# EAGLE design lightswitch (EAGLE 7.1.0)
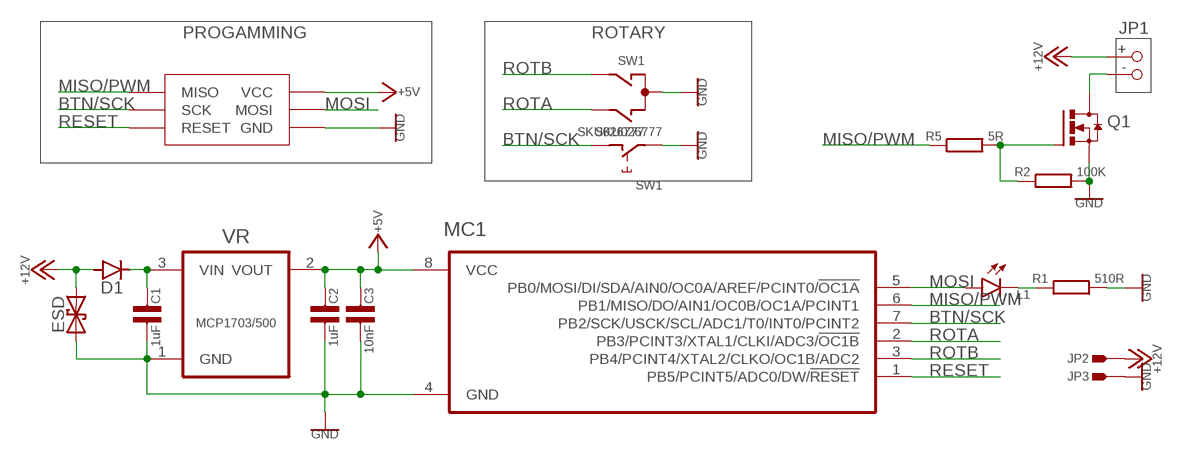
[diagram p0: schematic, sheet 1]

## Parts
C1  1uF  C-EU0603  [0603]
C2  1uF  C-EU0603  [0603]
C3  10nF  C-EU0603  [0603]
D1  DIODE0603  [0603-DIODE]
ESD  ESDSUPPRESSOR0603  [0603]
JP1  PINHD-1X2LED-STRIP  [CON-LEDSTRIP]
JP2  PINHD-1X11.5MM2  [1X01-HUGE]
JP3  PINHD-1X11.5MM2  [1X01-HUGE]
L1  LED0603  [0603-DIODE]
MC1  ATTINY85SOIC  [SOIC8-WIDE]
Q1  MOSFET-NCHSOT-23  [SOT23]
R1  510R  R-EU0603  [0603]
R2  100K  R-EU0603  [0603]
R5  5R  R-EU0603  [0603]
SW1  SKU026777  [SKU026777]
U$1  AVRISPTAG-CONNECT  [TAG-CONNECT-2030NL]
VR  MCP1703/500  MCP1703SOT23  [SOT23]

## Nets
+12V: D1.2(A) ESD.2 JP1.+ JP2.P$1
BTN/SCK: MC1.7(PB2/SCK/USCK/SCL/ADC1/T0/INT0/PCINT2) SW1.D U$1.3(SCK)
GND: C1.1 C2.1 C3.1 ESD.1 JP3.P$1 MC1.4(GND) Q1.2(S) R1.2 R2.2 SW1.C SW1.E U$1.6(GND) VR.1(GND)
MISO/PWM: MC1.6(PB1/MISO/DO/AIN1/OC0B/OC1A/PCINT1) R5.1 U$1.1(MISO)
MOSI: L1.2(A) MC1.5(PB0/MOSI/DI/SDA/AIN0/OC0A/AREF/PCINT0/!OC1A) U$1.4(MOSI)
N$1: C1.2 D1.1(K) VR.3(VIN)
N$2: L1.1(C) R1.1
OUT1: JP1.- Q1.3(D)
OWM: Q1.1(G) R2.1 R5.2
RESET: MC1.1(PB5/PCINT5/ADC0/DW/!RESET) U$1.5(RESET)
ROTA: MC1.2(PB3/PCINT3/XTAL1/CLKI/ADC3/!OC1B) SW1.B
ROTB: MC1.3(PB4/PCINT4/XTAL2/CLKO/OC1B/ADC2) SW1.A
VCC: C2.2 C3.2 MC1.8(VCC) U$1.2(VCC) VR.2(VOUT) ; supply symbol labelled +5V
Unconnected: SW1.GND1(G) SW1.GND2(G)

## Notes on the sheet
- PROGAMMING | ROTARY

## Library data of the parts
C1-C3 = MikesParts:C-EU
D1 = MikesParts:DIODE
ESD = MikesParts:ESDSUPPRESSOR: ESD Suppressor
JP1 = MikesParts:PINHD-1X2: PIN HEADER
JP2 JP3 = MikesParts:PINHD-1X1: PIN HEADER
L1 = MikesParts:LED: LED
MC1 = MikesParts:ATTINY85: 8-bit Microcontroller with In-System Programmable Flash; MPN: ATTINY85-20SU; OC_FARNELL: 1455164; OC_NEWARK: 58M3797; PACKAGE: SOIC-8; SUPPLIER: Atmel
Q1 = MikesParts:MOSFET-NCH: MOSFET N-Channel, eg BSS138, BUK7Y13, FDN335N
R1 R2 R5 = MikesParts:R-EU: resistor
SW1 = MikesParts:SKU026777: ALPS rotary Encoder EC12E series with switch; MPN: EC12E2424407; OC_FARNELL: 1520813; OC_NEWARK: 74M1068
U$1 = MikesParts:AVRISP
VR = MikesParts:MCP1703: IC REG LDO 250MA: 2V5, 3V3, 5V0

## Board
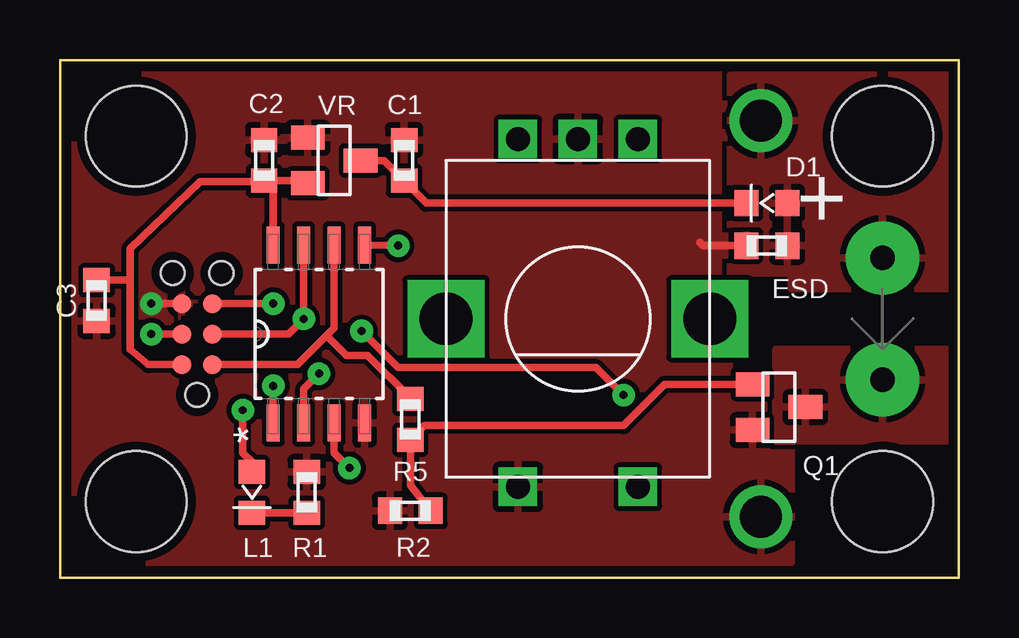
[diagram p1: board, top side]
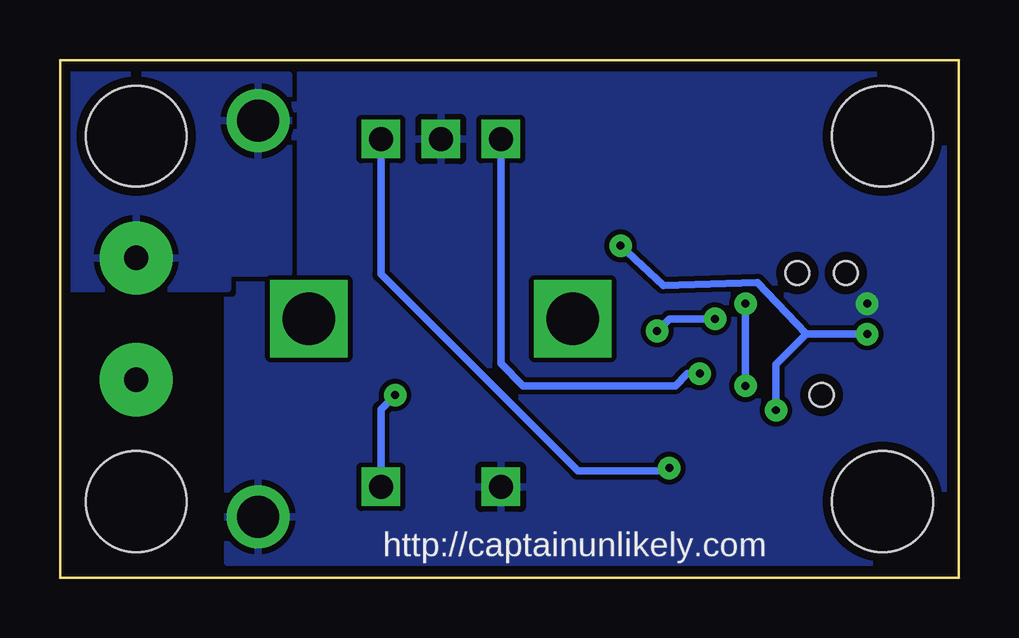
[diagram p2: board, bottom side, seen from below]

Size 37.47 x 21.59 mm. Coordinates in mm from the lower left corner, seen from the top.
Outline: 0,0 0,21.59 37.47,21.59 37.47,0 0,0
Copper layers (1*16): Top 0.0356mm / dielectric 1.5011mm / Bottom 0.0356mm
Design rules "default *": minimum track width 6mil, minimum drill 13mil, track to track 8mil, track to pad 8mil, pad to pad 8mil, via to via 8mil, smd to smd 8mil, copper to edge 15mil, drill to drill 6mil, minimum pad ring 12mil, minimum via ring 12mil, stop-mask expansion 4mil, vias tented up to drill 15mil, thermal gap 10mil
Holes 4.2 mm at 3.17,18.41 34.29,18.41 34.29,3.17 3.17,3.17

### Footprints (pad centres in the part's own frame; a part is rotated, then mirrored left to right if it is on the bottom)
0603 = smd 1 x 1.1: 1 -0.85,0; 2 0.85,0
0603-DIODE = smd 1 x 1.1: 1 -0.85,0; 2 0.85,0
CON-LEDSTRIP = drill 1.016 pad 3.048: + 0,-2.54; - 0,2.54
1X01-HUGE = drill 1.75: P$1 0,0
SOIC8-WIDE = smd 1.549 x 0.533: 1 -3.708,1.905; 2 -3.708,0.635; 3 -3.708,-0.635; 4 -3.708,-1.905; 5 3.708,-1.905; 6 3.708,-0.635; 7 3.708,0.635; 8 3.708,1.905
SOT23 = smd 1.4 x 1: 1 -1.1,0.95; 2 -1.1,-0.95; 3 1.1,0
SKU026777 = drill 1 square: A -2.5,-7.5; B 2.5,-7.5; C 0,-7.5; D -2.5,7; E 2.5,7 | drill 2.2 square: GND1 -5.5,0; GND2 5.5,0
TAG-CONNECT-2030NL = smd 0.787 x 0.787: 1 -1.27,-0.635; 2 -1.27,0.635; 3 0,-0.635; 4 0,0.635; 5 1.27,-0.635; 6 1.27,0.635 | hole 0.991: -2.54,0; 2.54,1.016; 2.54,-1.016

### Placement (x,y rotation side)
C1  14.35,17.4 270 top
C2  8.51,17.4 270 top
C3  1.52,11.56 90 top
D1  29.46,15.62 0 top
ESD  29.46,13.84 0 top
JP1  34.29,10.79 180 top
JP2  29.21,19.05 0 top
JP3  29.21,2.54 0 top
L1  8,3.56 90 top
MC1  10.79,10.16 90 top
Q1  29.97,7.11 0 top
R1  10.29,3.56 90 top
R2  14.61,2.79 180 top
R5  14.61,6.6 270 top
SW1  21.59,10.79 180 top
U$1  5.71,10.16 90 top
VR  11.43,17.4 0 top

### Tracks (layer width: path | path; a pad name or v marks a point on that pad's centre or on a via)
+12V
  pour Top: 27.94,20.95 27.94,12.7 30.48,12.7 30.48,12.06 37.47,12.06 37.47,20.95
  pour Bottom: 27.94,20.95 27.94,12.7 30.48,12.7 30.48,12.06 37.47,12.06 37.47,20.95
BTN/SCK  (via drill 0.33)
  Top 0.305: U$1.3 9.53,10.16 v10.16,10.79 MC1.7 | v23.5,7.62 22.35,8.76 14.1,8.76 v12.57,10.29
  Bottom 0.305: SW1.D 24.09,7.03 v23.5,7.62 | v10.16,10.79 12.06,10.79 v12.57,10.29
GND  (via drill 0.33)
  Top 0.305: U$1.6 v3.81,11.43 | ESD.1 26.8,13.84 26.67,13.97
  pour Top (rank 5): 0.64,20.95 0.64,0.64 30.48,0.64 30.48,20.95
  pour Bottom (rank 5): 0.64,20.95 0.64,0.64 30.48,0.64 30.48,20.95
MISO/PWM
  Top 0.305: U$1.1 9.91,8.89 11.11,10.1 | 11.11,10.1 11.43,10.41 MC1.6 | R5.1 14.61,7.49 12.83,9.27 11.94,9.27 11.11,10.1
MOSI  (via drill 0.33)
  Top 0.305: U$1.4 v3.81,10.16 | MC1.5 v14.1,13.84 | L1.2 8,4.83 7.62,5.21 v7.62,6.99
  Bottom 0.305: v3.81,10.16 6.35,10.16 | 6.35,10.16 8.38,12.32 12.32,12.19 v14.1,13.84 | 6.35,10.16 7.62,8.89 v7.62,6.99
N$1
  Top 0.305: D1.1 15.28,15.62 C1.2 13.5,17.4 VR.3
N$2
  Top 0.305: L1.1 R1.1
OUT1
  pour Top: 37.47,9.53 29.84,9.53 29.84,5.71 37.47,5.71
OWM
  Top 0.305: R2.1 14.61,3.85 R5.2 15.2,6.35 23.5,6.35 25.21,8.06 Q1.1
RESET  (via drill 0.33)
  Top 0.305: U$1.5 v8.89,11.43 | MC1.1 v8.89,8
  Bottom 0.305: v8.89,11.43 v8.89,8
ROTA  (via drill 0.33)
  Top 0.305: MC1.2 10.16,7.87 v10.79,8.51
  Bottom 0.305: v10.79,8.51 11.3,8.51 11.81,8 18.16,8 19.09,8.93 SW1.B
ROTB  (via drill 0.33)
  Top 0.305: MC1.3 11.43,5.21 v12.06,4.57
  Bottom 0.305: SW1.A 24.09,12.66 15.88,4.45 12.19,4.45 v12.06,4.57
VCC
  Top 0.305: U$1.2 3.68,8.89 2.92,9.53 2.92,12.7 | 2.92,12.7 2.92,13.72 5.84,16.51 8.47,16.51 C2.2 | C2.2 10.23,16.55 VR.2 | MC1.8 8.89,16.51 8.55,16.51 C2.2 | C3.2 2.92,12.41 2.92,12.7

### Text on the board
tNames: +
bNames: http://captainunlikely.com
